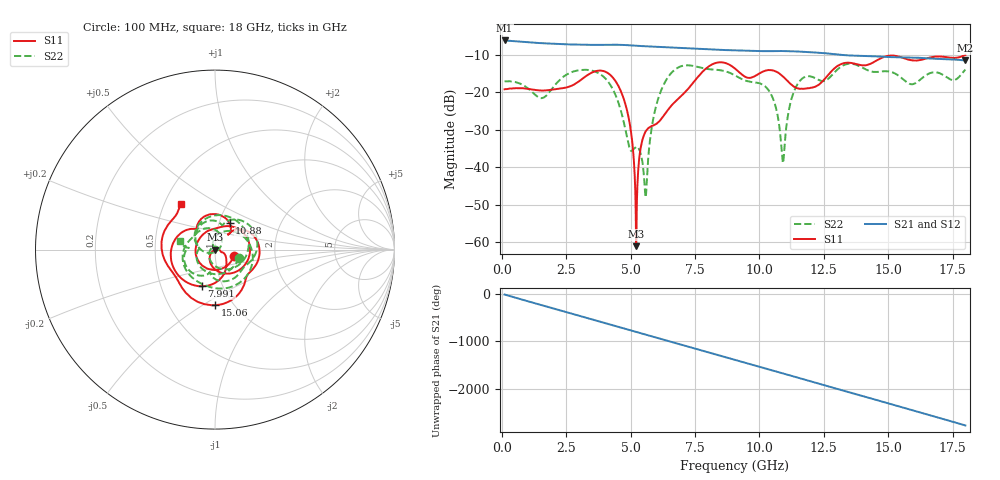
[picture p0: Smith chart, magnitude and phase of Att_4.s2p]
#  HZ  S  DB  R  50.00
! Rohde & Schwarz Vector Network Analyzer
! Rohde-Schwarz,ZNB40-4Port,1311601084101679,3.45
! Created: UTC 4/25/2025, 8:44:19 AM
! freq[Hz]  db:S11  ang:S11  db:S21  ang:S21  db:S12  ang:S12  db:S22  ang:S22
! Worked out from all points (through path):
!   1750 points, 100 MHz to 18 GHz, reference 50 ohm
!   highest |S21| = -6.13 dB at 100 MHz (marker M1); lowest = -11.5 dB at 18 GHz (marker M2)
!   group delay of S21, straight-line fit = 427 ps
!   lowest |S11| = -61.1 dB at 5.207 GHz (marker M3), VSWR 1.00, Z = 50 - j0.0817 ohm
!   |S11| at or under -10 dB: start of sweep to end of sweep
!   |S22| runs from -48.1 to -12.3 dB; largest |S21 - S12| = 0.00054
!   S11 on the Smith chart (normalised r, x): 100 MHz: 1.23, -0.09; 7.991 GHz: 0.80, -0.34; 10.88 GHz: 1.12, +0.34; 15.06 GHz: 0.83, -0.57; 18 GHz: 0.61, +0.34
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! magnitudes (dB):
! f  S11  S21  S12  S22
! 100 MHz  -19.2  -6.1  -6.1  -17.0
! 1.553 GHz  -19.5  -6.9  -6.9  -21.5
! 3.088 GHz  -16.6  -7.3  -7.3  -14.0
! 3.969 GHz  -14.4  -7.3  -7.3  -16.0
! 4.562 GHz  -18.9  -7.3  -7.3  -23.6
! 4.972 GHz  -28.8  -7.4  -7.4  -35.2
! 5.207 GHz  -61.1  -7.5  -7.5  -34.6
! 5.391 GHz  -34.7  -7.6  -7.6  -36.5
! 5.586 GHz  -30.4  -7.7  -7.7  -47.9
! 5.811 GHz  -29.0  -7.8  -7.8  -29.6
! 6.067 GHz  -28.0  -7.8  -7.8  -21.7
! 6.804 GHz  -22.0  -8.1  -8.1  -13.5
! 7.991 GHz  -13.3  -8.5  -8.5  -13.8
! 9.055 GHz  -13.7  -8.8  -8.8  -15.5
! 10.4 GHz  -14.1  -9.0  -9.0  -19.9
! 10.67 GHz  -14.6  -9.0  -9.0  -25.0
! 10.88 GHz  -15.5  -9.0  -9.0  -36.9
! 11.36 GHz  -18.5  -9.0  -9.0  -19.5
! 12.04 GHz  -18.7  -9.3  -9.3  -15.9
! 15.02 GHz  -10.2  -10.6  -10.6  -14.4
! 15.06 GHz  -10.2  -10.6  -10.6  -14.5
! 18 GHz  -10.0  -11.5  -11.5  -13.9
